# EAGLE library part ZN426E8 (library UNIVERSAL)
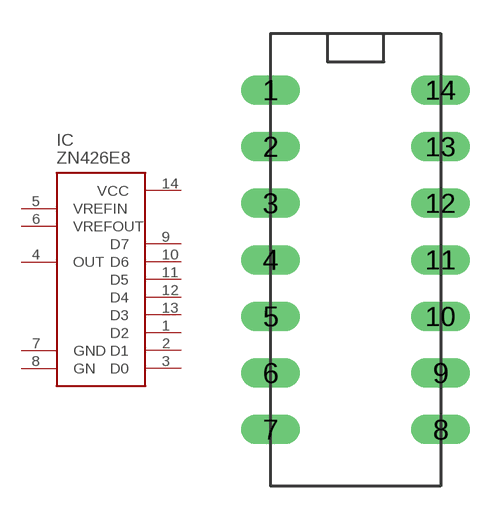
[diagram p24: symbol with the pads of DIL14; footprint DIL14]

Designator prefix IC

## ZN426E8  [DIL14]
1  D2  in
2  D1  in
3  D0  in
4  OUT  out
5  VREFIN  in
6  VREFOUT  sup
7  GND  sup
8  GN  sup
9  D7  in
10  D6  in
11  D5  in
12  D4  in
13  D3  in
14  VCC  sup

## Footprint DIL14 (pad centres in mm)
drill 0.813 pad 1.092 long: 1 0,0; 2 0,-2.54; 3 0,-5.08; 4 0,-7.62; 5 0,-10.16; 6 0,-12.7; 7 0,-15.24; 8 7.62,-15.24; 9 7.62,-12.7; 10 7.62,-10.16; 11 7.62,-7.62; 12 7.62,-5.08; 13 7.62,-2.54; 14 7.62,0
